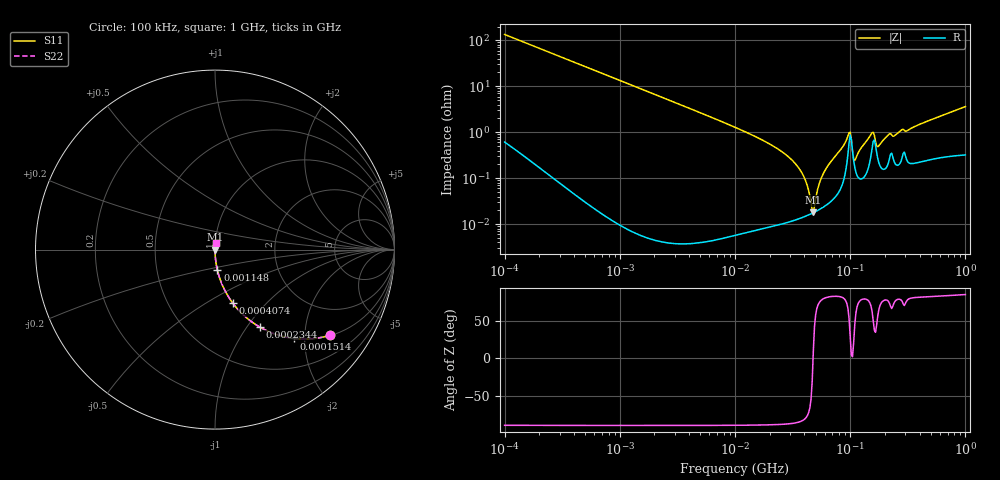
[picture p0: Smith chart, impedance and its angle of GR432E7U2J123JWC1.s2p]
!Murata Part Number: GR432E7U2J123JWC1
!These Parameters are Measured in Series Mode Connection
!Data Generated on Jun 10, 2025
!  o--ll--o
!Port1  Port2
!  o------o
!Operation Temp=25[degC], DC Bias Voltage=0[V]
!Freq. Start=100[kHz] Stop=1000[MHz] 401[Steps]
# Hz S RI R 50
!Freq.(Hz) S11(Real) S11(Imag) S21(Real) S21(Imag) S12(Real) S12(Imag) S22(Real) S22(Imag)
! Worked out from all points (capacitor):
!   401 points, 100 kHz to 1 GHz, reference 50 ohm
!   read as one part in series: C = 11.8 nF near 104.7 kHz
!   lowest |Z| = 18 mohm at 47.86 MHz (marker M1)
!   series resonance near 47.63 MHz, so ESL is about 940 pH
!   S11 on the Smith chart (normalised r, x): 100 kHz: 1.01, -2.69; 151.4 kHz: 1.01, -1.78; 234.4 kHz: 1.00, -1.15; 407.4 kHz: 1.00, -0.66; 1.148 MHz: 1.00, -0.23; 1 GHz: 1.01, +0.07
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100000  0.6426 -0.4769  0.3574 0.4769  0.3574 0.4769  0.6426 -0.4769
151356  0.4411 -0.4949  0.5589 0.4949  0.5589 0.4949  0.4411 -0.4949
234423  0.248 -0.4308  0.752 0.4308  0.752 0.4308  0.248 -0.4308
407380  0.0986 -0.2974  0.9014 0.2974  0.9014 0.2974  0.0986 -0.2974
467735  0.0766 -0.2654  0.9234 0.2654  0.9234 0.2654  0.0766 -0.2654
1148154  0.0136 -0.1155  0.9864 0.1155  0.9864 0.1155  0.0136 -0.1155
2187762  0.00379 -0.0611  0.9962 0.0611  0.9962 0.0611  0.00379 -0.0611
1e7  0.000222 -0.0128  0.9998 0.0128  0.9998 0.0128  0.000222 -0.0128
2.089296e7  0.000116 -0.00521  0.9999 0.00521  0.9999 0.00521  0.000116 -0.00521
3.162278e7  0.000124 -0.00241  0.9999 0.00241  0.9999 0.00241  0.000124 -0.00241
3.981072e7  0.000146 -0.00104  0.9999 0.00104  0.9999 0.00104  0.000146 -0.00104
4.677351e7  0.000173 -0.000106  0.9998 0.000106  0.9998 0.000106  0.000173 -0.000106
4.786301e7  0.000178 2.87e-05  0.9998 -2.87e-05  0.9998 -2.87e-05  0.000178 2.87e-05
5.888437e7  0.00024 0.00129  0.9998 -0.00129  0.9998 -0.00129  0.00024 0.00129
9.549926e7  0.0033 0.00754  0.9967 -0.00754  0.9967 -0.00754  0.0033 0.00754
1e8  0.00872 0.00474  0.9913 -0.00474  0.9913 -0.00474  0.00872 0.00474
1.071519e8  0.00243 0.000915  0.9976 -0.000915  0.9976 -0.000915  0.00243 0.000915
1.122018e8  0.00135 0.00239  0.9987 -0.00239  0.9987 -0.00239  0.00135 0.00239
1.513561e8  0.00314 0.00835  0.9969 -0.00835  0.9969 -0.00835  0.00314 0.00835
1.778279e8  0.00214 0.00467  0.9979 -0.00467  0.9979 -0.00467  0.00214 0.00467
2.187762e8  0.00267 0.00879  0.9973 -0.00879  0.9973 -0.00879  0.00267 0.00879
1e9  0.00449 0.0358  0.9955 -0.0358  0.9955 -0.0358  0.00449 0.0358
